PROGRAM RobotMove //基本运动控制,为了便于调试机器人及9点标定
VAR 
	//正反向点动
	FB_RobotJog      : ARRAY[1..4] OF MC_Jog;
	b_JogFw          : ARRAY[1..4] OF BOOL;           
	b_JogBw          : ARRAY[1..4] OF BOOL;
	
	//绝对定位
	FB_MoveAB        : ARRAY[1..4] OF MC_MoveAbsolute;
	b_StartMove      : ARRAY[1..4] OF BOOL;
	MovePosition     : ARRAY[1..4] OF LREAL;             //定义绝对定位位置
	MoveVelo         : ARRAY[1..4] OF LREAL;             //定义绝对定位速度
	FB_MoveModule    : MC_MoveModulo;
END_VAR

MotionCommand();//调用运动控制功能块

ACTION MotionCommand:
//C轴（旋转轴）点动
FB_RobotJog[1](
	Axis:=AxisArray[4] , 
	JogForward:=b_JogFw[1] , 
	JogBackwards:=b_JogBw[1], 
	Mode:=MC_JOGMODE_STANDARD_FAST , 
);

//X轴点动
FB_RobotJog[2](
	Axis:=AxisArray[5] , 
	JogForward:=b_JogFw[2] , 
	JogBackwards:=b_JogBw[2], 
	Mode:=MC_JOGMODE_STANDARD_FAST , 
);

//Y轴点动
FB_RobotJog[3](
	Axis:=AxisArray[6] , 
	JogForward:=b_JogFw[3] , 
	JogBackwards:=b_JogBw[3], 
	Mode:=MC_JOGMODE_STANDARD_FAST , 
);

//Z轴点动
FB_RobotJog[4](
	Axis:=AxisArray[7] , 
	JogForward:=b_JogFw[4] , 
	JogBackwards:=b_JogBw[4], 
	Mode:=MC_JOGMODE_STANDARD_FAST , 
);

//C轴绝对定位
FB_MoveModule(
	Axis:=AxisArray[4] , 
	Execute:=b_StartMove[1] , 
	Position:=MovePosition[1] , 
	Velocity:=MoveVelo[1] , 
);

//X轴绝对定位
FB_MoveAB[2](
	Axis:=AxisArray[5] , 
	Execute:=b_StartMove[2] , 
	Position:=MovePosition[2] , 
	Velocity:=MoveVelo[2] , 
);

//Y轴绝对定位
FB_MoveAB[3](
	Axis:=AxisArray[6] , 
	Execute:=b_StartMove[3] , 
	Position:=MovePosition[3] , 
	Velocity:=MoveVelo[3] , 
);

//Z轴绝对定位
FB_MoveAB[4](
	Axis:=AxisArray[7] , 
	Execute:=b_StartMove[4] , 
	Position:=MovePosition[4] , 
	Velocity:=MoveVelo[4] , 
);
END_ACTION

END_PROGRAM
